(* Logix 5000 AddOnInstructionDefinition export AMCI_SMD23E2_Reset_Errors; software revision 20.03 *)

ADD_ON_INSTRUCTION AMCI_SMD23E2_Reset_Errors   (* revision 1.0, vendor AMCI *)
VAR_IN_OUT
   AMCI_SMD23E2_output_data : _000A:SMD23E2_788832CB:O:0; {required}
END_VAR
VAR
   command_data_block : INT[10];
        [0]   // Command Bits MSW
        [1]   // Command Bits LSW
        [2]   // Upper Target Position
        [3]   // Lower Target Position
        [4]   // Upper Programmed Speed
        [5]   // Lower Programmed Speed
END_VAR

ROUTINE Logic   (* ladder *)
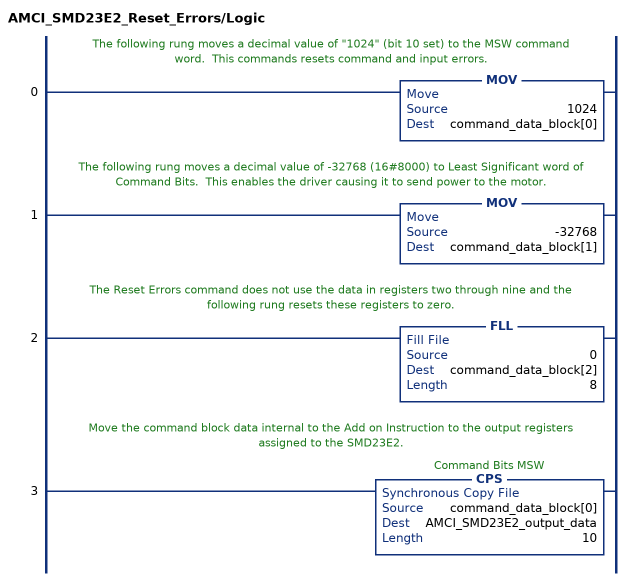
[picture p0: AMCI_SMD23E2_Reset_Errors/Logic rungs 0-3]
   // The following rung moves a decimal value of "1024" (bit 10 set) to the MSW command word.  This commands resets command and input errors.
   0: MOV(1024,command_data_block[0]);
   // The following rung moves a decimal value of -32768 (16#8000) to Least Significant word of Command Bits.  This enables the driver causing it to send power to the motor.
   1: MOV(-32768,command_data_block[1]);
   // The Reset Errors command does not use the data in registers two through nine and the following rung resets these registers to zero.
   2: FLL(0,command_data_block[2],8);
   // Move the command block data internal to the Add on Instruction to the output registers assigned to the SMD23E2.
   3: CPS(command_data_block[0],AMCI_SMD23E2_output_data,10);
END_ROUTINE
END_ADD_ON_INSTRUCTION
